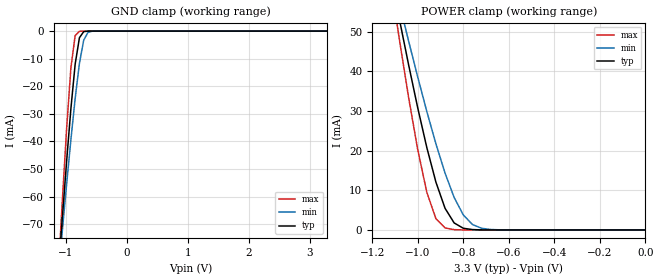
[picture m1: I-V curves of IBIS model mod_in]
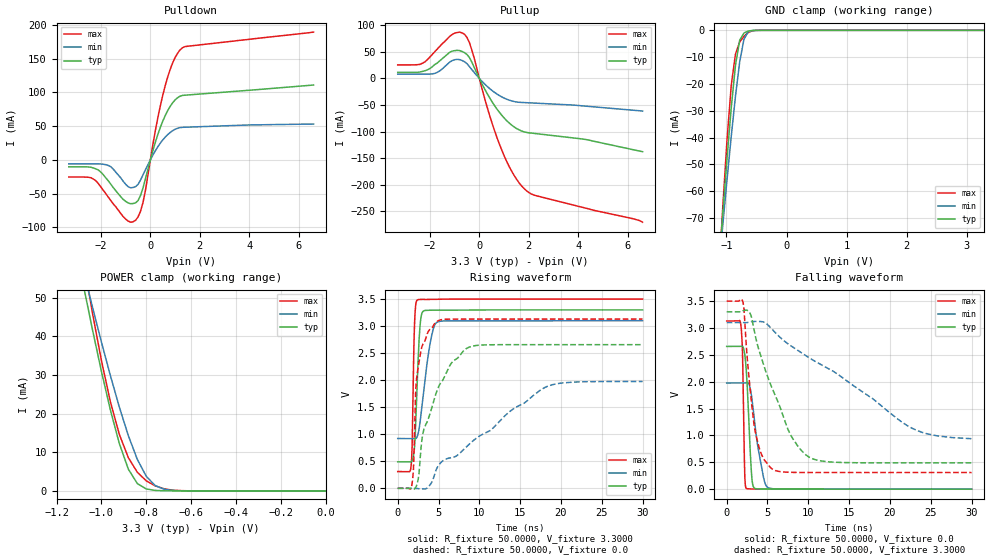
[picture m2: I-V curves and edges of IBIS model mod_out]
| IBIS (I/O, Buffer, Information, Specification) Model, officially
| electronic behavioral standard for Buffer structures of digital pins.
[IBIS ver]  4.0
[File name] 54ac16244_3v1_3v5_rev1.ibs
[File Rev]  1.0
[Date]   19 June 2020
[Source]   CAD & Design Services (Catania) - STMicroelectronics
[Notes]
  (Note1) This IBIS model is the model of the product with package
   (Flat48 package elements);
  (Note2) This IBIS model is extracted with nominal 3.3V power supply
   (min:3.1V, typ:3.3V, max:3.5V);
  (Note3) This model has few Warnings about the non-monotonicity
   of I-V curves, but they are not indicative of problems
   inside the model;
[Copyright] (c) 2020 STMicroelectronics
|   Component 54AC16244
[Component] 54AC16244
[Manufacturer] STMicroelectronics
[Package]
| variable   typ   min   max
R_pkg   0.0   0.0   0.0
L_pkg   0.0H   0.0H   0.0H
C_pkg   0.0F   0.0F   0.0F
[Pin]  signal_name   model_name   R_pin   L_pin   C_pin
1   N1GN   mod_in   467.00m   6.34nH   1.49pF
2   N1Y1   mod_out   467.00m   6.34nH   1.49pF
3   N1Y2   mod_out   467.00m   6.34nH   1.49pF
4   GND1   GND   467.00m   6.34nH   1.49pF
5   N1Y3   mod_out   145.00m   3.32nH   1.24pF
6   N1Y4   mod_out   141.00m   2.11nH   1.24pF
7   VCC1   POWER   141.00m   2.11nH   1.24pF
8   N2Y1   mod_out   141.00m   2.11nH   1.24pF
9   N2Y2   mod_out   141.00m   2.11nH   1.24pF
10   GND2   GND   141.00m   2.11nH   1.24pF
11   N2Y3   mod_out   141.00m   2.11nH   1.24pF
12   N2Y4   mod_out   141.00m   2.11nH   1.24pF
13   N3Y1   mod_out   141.00m   2.11nH   1.24pF
14   N3Y2   mod_out   141.00m   2.11nH   1.24pF
15   GND3   GND   141.00m   2.11nH   1.24pF
16   N3Y3   mod_out   141.00m   2.11nH   1.24pF
17   N3Y4   mod_out   141.00m   2.11nH   1.24pF
18   VCC2   POWER   141.00m   2.11nH   1.24pF
19   N4Y1   mod_out   141.00m   2.11nH   1.24pF
20   N4Y2   mod_out   145.00m   3.32nH   1.24pF
21   GND4   GND   467.00m   6.34nH   1.49pF
22   N4Y3   mod_out   467.00m   6.34nH   1.49pF
23   N4Y4   mod_out   467.00m   6.34nH   1.49pF
24   N4GN   mod_in   467.00m   6.34nH   1.49pF
25   N3GN   mod_in   467.00m   6.34nH   1.49pF
26   N4A4   mod_in   467.00m   6.34nH   1.49pF
27   N4A3   mod_in   467.00m   6.34nH   1.49pF
28   GND5   GND   467.00m   6.34nH   1.49pF
29   N4A2   mod_in   145.00m   3.32nH   1.24pF
30   N4A1   mod_in   141.00m   2.11nH   1.24pF
31   VCC3   POWER   141.00m   2.11nH   1.24pF
32   N3A4   mod_in   141.00m   2.11nH   1.24pF
33   N3A3   mod_in   141.00m   2.11nH   1.24pF
34   GND6   GND   141.00m   2.11nH   1.24pF
35   N3A2   mod_in   141.00m   2.11nH   1.24pF
36   N3A1   mod_in   141.00m   2.11nH   1.24pF
37   N2A4   mod_in   141.00m   2.11nH   1.24pF
38   N2A3   mod_in   141.00m   2.11nH   1.24pF
39   GND7   GND   141.00m   2.11nH   1.24pF
40   N2A2   mod_in   141.00m   2.11nH   1.24pF
41   N2A1   mod_in   141.00m   2.11nH   1.24pF
42   VCC4   POWER   141.00m   2.11nH   1.24pF
43   N1A4   mod_in   141.00m   2.11nH   1.24pF
44   N1A3   mod_in   145.00m   3.32nH   1.24pF
45   GND8   GND   467.00m   6.34nH   1.49pF
46   N1A2   mod_in   467.00m   6.34nH   1.49pF
47   N1A1   mod_in   467.00m   6.34nH   1.49pF
48   N2GN   mod_in   467.00m   6.34nH   1.49pF
| Models and submodels in the file (2): mod_in (Input), mod_out (3-state)
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|   Model mod_in
[Model]   mod_in
Model_type Input
Vinl   =   1.000V
Vinh   =   2.300V
C_comp   0.584pF   0.464pF   0.735pF
[Temperature Range]  25.0000   85.0000   -35.0000
[Voltage Range]   3.3000V   3.1000V   3.5000V
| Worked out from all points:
|   GND clamp passes 1 mA (typ) near -0.74 V on its own axis
|   POWER clamp passes 1 mA (typ) near -0.82 V on its own axis
[GND_clamp]
|Voltage   I(typ)   I(min)   I(max)
-3.3V     -798.8mA   -660.7mA   -1.026A
-1.13V    -88.7mA    -89.38mA   -88.86mA
-1.06V    -67.54mA   -72.2mA    -61.29mA
-990mV    -47.13mA   -55.44mA   -35.35mA
-920mV    -28.09mA   -39.35mA   -13.3mA
-850mV    -11.96mA   -24.39mA   -1.606mA
-780mV    -2.392mA   -11.63mA   -63.06uA
-710mV    -202.9uA   -3.285mA   -2.096uA
-640mV    -13.61uA   -477.6uA   -69.21nA
-570mV    -893.7nA   -52.07uA   -2.293nA
3.28V     6.52pA     19.08pA    6.12pA
[POWER_clamp]
|Voltage   I(typ)   I(min)   I(max)
-3.28V    769.1mA    633mA      992.8mA
-1.12V    64.69mA    66.5mA     63mA
-1.08V    52.98mA    56.96mA    47.82mA
-1.04V    41.63mA    47.62mA    33.4mA
-1V       30.8mA     38.55mA    20.27mA
-960mV    20.77mA    29.86mA    9.49mA
-920mV    12.05mA    21.7mA     2.829mA
-880mV    5.461mA    14.34mA    521.7uA
-840mV    1.772mA    8.192mA    78.11uA
-800mV    437uA      3.801mA    11.21uA
-720mV    20.4uA     427.9uA    227.5nA
0V        6.6pA      7.017pA    7pA
|   Model mod_out
[Model]   mod_out
Model_type 3-state
Polarity   Non-Inverting
Enable   Active-Low
Vmeas  =   1.650V
Cref   =   50pF
Rref   =   500
C_comp   3.063pF   2.433pF   4.038pF
[Temperature Range]  25.0000   85.0000   -35.0000
[Voltage Range]   3.3000V   3.1000V   3.5000V
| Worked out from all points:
|   slope of the pulldown table from 0 to 0.495 V, typ, clamps not added: 8.73 ohm
|   slope of the pullup table from 0 to 0.495 V, typ, clamps not added: 11.6 ohm
|   GND clamp passes 1 mA (typ) near -0.71 V on its own axis
|   POWER clamp passes 1 mA (typ) near -0.81 V on its own axis
|   rising waveform, R_fixture 50.0000, V_fixture 3.3000: 20-80 % time 452ps typ, 1.11ns min, 235ps max; typ from 0.489 V to 3.3 V
|   rising waveform, R_fixture 50.0000, V_fixture 0.0: 20-80 % time 3.19ns typ, 10.7ns min, 798ps max; typ from 0 V to 2.66 V
|   falling waveform, R_fixture 50.0000, V_fixture 0.0: 20-80 % time 502ps typ, 1.12ns min, 219ps max; typ from 2.66 V to 0 V
|   falling waveform, R_fixture 50.0000, V_fixture 3.3000: 20-80 % time 4.01ns typ, 12.5ns min, 1.36ns max; typ from 3.3 V to 0.489 V
[Pulldown]
|Voltage   I(typ)   I(min)   I(max)
-3.3V     -10.36mA   -6mA       -25.42mA
-2.3V     -12.22mA   -6mA       -28.55mA
-1.6V     -36.13mA   -10.2mA    -60.32mA
-1.1V     -58.64mA   -31.7mA    -84.14mA
-700mV    -64.74mA   -41mA      -91.85mA
-500mV    -60.41mA   -36.43mA   -84.71mA
-300mV    -41.86mA   -22.4mA    -63.42mA
200mV     25.93mA    13.4mA     42.97mA
600mV     65.52mA    33.66mA    109.9mA
900mV     84.46mA    43.14mA    143.5mA
1.2V      94.2mA     47.71mA    162.8mA
6.6V      110.8mA    53mA       189.2mA
[Pullup]
|Voltage   I(typ)   I(min)   I(max)
-3.3V     11.36mA    8mA        25.42mA
-2.3V     13.22mA    8mA        28.55mA
-1.7V     29.13mA    11.44mA    55.32mA
-1.1V     51.31mA    33.42mA    82.6mA
-600mV    48.64mA    31.41mA    83.21mA
-300mV    30.29mA    16.47mA    52.93mA
300mV     -27.16mA   -14.22mA   -51.55mA
800mV     -63.16mA   -31.98mA   -122.3mA
1.3V      -87.59mA   -42.29mA   -174.1mA
1.8V      -100.5mA   -45.44mA   -206.9mA
2.3V      -104mA     -46.62mA   -220.9mA
6.6V      -138mA     -61.5mA    -270.7mA
[GND_clamp]
|Voltage   I(typ)   I(min)   I(max)
-3.3V     -798.9mA   -660.7mA   -1.027A
-1.13V    -89mA      -89.44mA   -92.29mA
-1.06V    -67.9mA    -72.26mA   -65.42mA
-990mV    -47.6mA    -55.52mA   -40.63mA
-920mV    -28.75mA   -39.44mA   -20.38mA
-850mV    -12.97mA   -24.5mA    -8.814mA
-780mV    -3.71mA    -11.77mA   -4.375mA
-710mV    -1.021mA   -3.418mA   -2.22mA
-640mV    -262.7uA   -547.4uA   -880.2uA
-570mV    -57.33uA   -75.33uA   -168.7uA
-500mV    -11.95uA   -12.06uA   -22.88uA
3.28V     84.16pA    386.4pA    18.43pA
[POWER_clamp]
|Voltage   I(typ)   I(min)   I(max)
-3.28V    769.1mA    633mA      996mA
-1.08V    53.09mA    56.93mA    59.55mA
-1.04V    41.75mA    47.59mA    46.05mA
-1V       30.94mA    38.52mA    33.73mA
-960mV    20.93mA    29.82mA    23.07mA
-920mV    12.22mA    21.66mA    14.6mA
-880mV    5.633mA    14.3mA     8.599mA
-840mV    1.905mA    8.154mA    4.827mA
-800mV    513.7uA    3.769mA    2.605mA
-760mV    132.7uA    1.374mA    1.301mA
-720mV    36.81uA    421.8uA    534uA
0V        86.27pA    276pA      0A
[Ramp]
| variable   typ   min   max
dV/dt_r  1.5938/3.1727n   1.1861/10.4720n   1.8780/0.8871n
dV/dt_f  1.6861/4.0132n   1.2977/12.5069n   1.9142/1.3588n
R_load = 50.0000
[Rising Waveform]
R_fixture= 50.0000
V_fixture= 3.3000
V_fixture_min= 3.1000
V_fixture_max= 3.5000
|time   V(typ)   V(min)   V(max)
0s        489.4mV    920.1mV    309.5mV
1.65ns    489mV      920.5mV    428.9mV
1.77ns    512.3mV    920.6mV    809.8mV
2.07ns    784.8mV    915.9mV    3.079V
2.37ns    1.892V     951.2mV    3.48V
2.67ns    2.875V     1.148V     3.492V
2.91ns    3.209V     1.447V     3.494V
3.93ns    3.293V     2.648V     3.495V
4.83ns    3.296V     3.073V     3.496V
30ns      3.3V       3.1V       3.5V
[Rising Waveform]
R_fixture= 50.0000
V_fixture= 0.0
V_fixture_min= 0.0
V_fixture_max= 0.0
|time   V(typ)   V(min)   V(max)
0s        132.2pV    219.5pV    86.68pV
1.68ns    -4.553mV   28.64uV    25.31mV
1.92ns    -13.04mV   588.6uV    340.2mV
2.19ns    10.25mV    -1.402mV   1.754V
2.43ns    114.9mV    -6.009mV   2.159V
3.09ns    1.016V     -12.03mV   2.665V
4.83ns    1.813V     380.2mV    3.089V
9.27ns    2.633V     883.9mV    3.13V
18.42ns   2.657V     1.891V     3.13V
30ns      2.657V     1.976V     3.13V
[Falling Waveform]
R_fixture= 50.0000
V_fixture= 0.0
V_fixture_min= 0.0
V_fixture_max= 0.0
|time   V(typ)   V(min)   V(max)
0s        2.657V     1.976V     3.13V
1.74ns    2.656V     1.975V     3.055V
1.92ns    2.663V     1.975V     2.633V
2.22ns    2.5V       1.977V     232.8mV
2.4ns     2.219V     1.982V     15.32mV
3.06ns    255.5mV    1.72V      3.574mV
3.42ns    17.11mV    1.254V     2.441mV
4.53ns    2.832mV    208.6mV    1.899mV
5.22ns    1.828mV    20.28mV    2.08mV
30ns      -218.4nV   76.56uV    -762.9nV
[Falling Waveform]
R_fixture= 50.0000
V_fixture= 3.3000
V_fixture_min= 3.1000
V_fixture_max= 3.5000
|time   V(typ)   V(min)   V(max)
0s        3.3V       3.1V       3.5V
2.01ns    3.32V      3.1V       3.472V
2.73ns    3.304V     3.111V     2.084V
3.45ns    2.894V     3.122V     1.108V
4.35ns    2.398V     3.117V     617.4mV
5.55ns    1.885V     2.979V     377.9mV
8.01ns    961.8mV    2.655V     312.5mV
10.68ns   557.4mV    2.393V     309.6mV
22.68ns   489.4mV    1.137V     309.5mV
30ns      489.4mV    939.4mV    309.5mV
